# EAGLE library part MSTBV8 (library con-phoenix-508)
PHOENIX
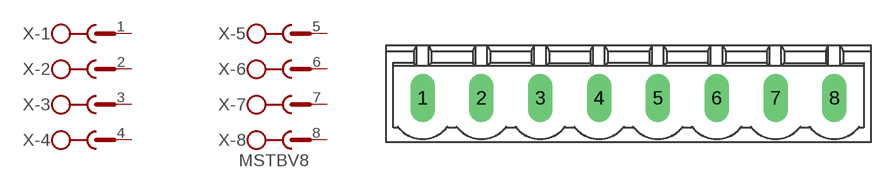
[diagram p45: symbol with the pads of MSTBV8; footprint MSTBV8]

Designator prefix X; gates -1=SK -2=SK -3=SK -4=SK -5=SK -6=SK -7=SK -8=SKV

## MSTBV8 (MPN: MSTBV 2,5/8-GF-5.08; OC_FARNELL: 1792797; OC_NEWARK: 69R9850)  [MSTBV8]
1  -1:1  pas
2  -2:1  pas
3  -3:1  pas
4  -4:1  pas
5  -5:1  pas
6  -6:1  pas
7  -7:1  pas
8  -8:1  pas

## Footprint MSTBV8 (pad centres in mm)
PHOENIX
drill 1.397 long: 1 -17.78,0; 2 -12.7,0; 3 -7.62,0; 4 -2.54,0; 5 2.54,0; 6 7.62,0; 7 12.7,0; 8 17.78,0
